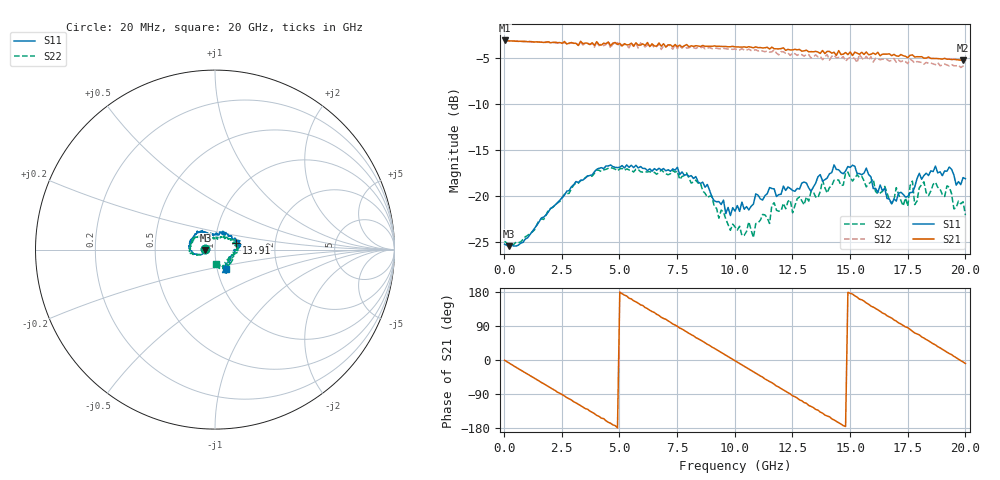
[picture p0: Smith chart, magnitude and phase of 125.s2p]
!Agilent Technologies,N5230A,US43500223,A.07.50.48
!Agilent N5230A: A.07.50.48
!Date: Thursday, October 08, 2015 17:00:51
!Correction: S11(Full 2 Port(1,2))
!S21(Full 2 Port(1,2))
!S12(Full 2 Port(1,2))
!S22(Full 2 Port(1,2))
!S2P File: Measurements: S11, S21, S12, S22:
# Hz S  RI  R 50
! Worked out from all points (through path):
!   201 points, 20 MHz to 20 GHz, reference 50 ohm
!   highest |S21| = -3.15 dB at 20 MHz (marker M1); lowest = -5.3 dB at 19.9 GHz (marker M2)
!   group delay of S21, straight-line fit = 101 ps
!   lowest |S11| = -25.4 dB at 219.8 MHz (marker M3), VSWR 1.11, Z = 44.9 - j0.152 ohm
!   |S11| at or under -10 dB: start of sweep to end of sweep
!   |S22| runs from -25.3 to -16.9 dB; largest |S21 - S12| = 0.081
!   S11 on the Smith chart (normalised r, x): 20 MHz: 0.90, +0.00; 13.91 GHz: 1.26, +0.10; 20 GHz: 1.10, -0.24
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2e7  -0.0549 0.00136  0.6956 -0.00959  0.6948 -0.0104  -0.0569 0.00142
2.198e8  -0.0535 -0.00168  0.6846 -0.1001  0.684 -0.1007  -0.0546 -0.00166
1.9181e9  -0.0772 -0.0279  0.2316 -0.6438  0.2228 -0.642  -0.0795 -0.027
2.6174e9  -0.098 -0.0254  -0.0601 -0.6842  -0.0691 -0.6735  -0.0978 -0.0304
3.4166e9  -0.1204 -0.0209  -0.3755 -0.5521  -0.3899 -0.529  -0.1191 -0.0262
4.9151e9  -0.1407 0.0225  -0.662 -0.0103  -0.6771 0.0219  -0.1366 0.0085
5.7143e9  -0.1373 0.0516  -0.6046 0.3021  -0.595 0.3244  -0.1371 0.0267
6.7133e9  -0.1129 0.0851  -0.3122 0.5974  -0.2841 0.6014  -0.1256 0.0465
8.1119e9  -0.0784 0.1024  0.2544 0.5991  0.2785 0.581  -0.0953 0.0687
9.1109e9  -0.0417 0.0844  0.5573 0.3342  0.5567 0.2983  -0.0557 0.0678
1.001e10  0.00241 0.0828  0.6416 -0.0238  0.6229 -0.0549  -0.0311 0.0606
1.08092e10  0.0248 0.087  0.541 -0.3321  0.5054 -0.3466  0.0137 0.058
1.17083e10  0.0538 0.0952  0.276 -0.5632  0.238 -0.5701  0.049 0.0778
1.26074e10  0.0758 0.0743  -0.0736 -0.6188  -0.113 -0.5784  0.0579 0.0668
1.34066e10  0.0931 0.0618  -0.3503 -0.492  -0.3477 -0.4456  0.0903 0.0541
1.39061e10  0.116 0.0393  -0.4845 -0.3379  -0.4685 -0.3209  0.104 0.0388
1.54046e10  0.1312 0.0173  -0.5519 0.1951  -0.5474 0.2064  0.126 0.00288
1.67033e10  0.0891 -0.0363  -0.2354 0.5395  -0.1955 0.5008  0.0892 -0.0339
1.8002e10  0.0617 -0.1176  0.2277 0.5198  0.2538 0.467  0.0832 -0.0735
1.91009e10  0.0684 -0.1182  0.5061 0.2313  0.4828 0.1882  0.0456 -0.0883
1.99001e10  0.0669 -0.1065  0.5397 -0.0501  0.5004 -0.071  0.014 -0.092
2e10  0.0612 -0.108  0.5365 -0.0857  0.4985 -0.1124  0.00674 -0.0785
